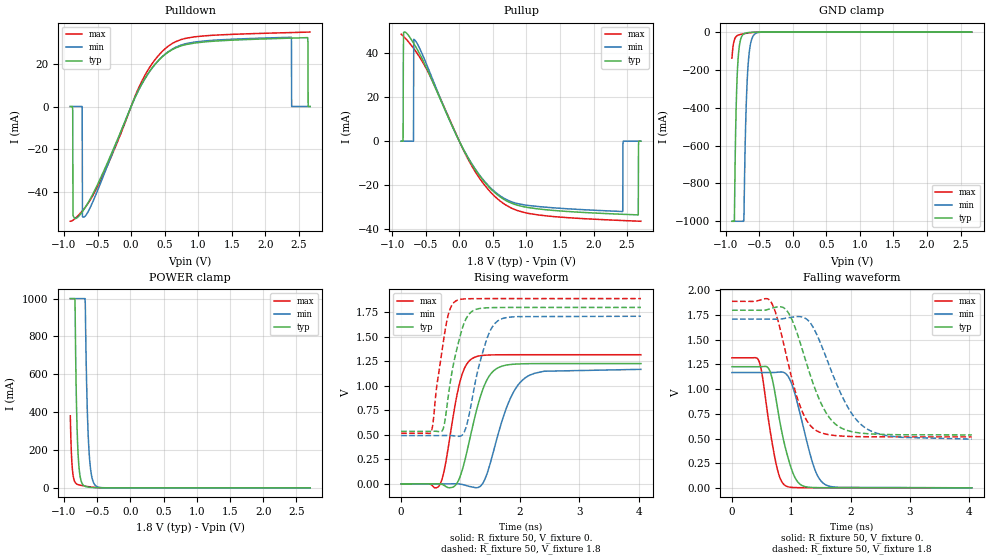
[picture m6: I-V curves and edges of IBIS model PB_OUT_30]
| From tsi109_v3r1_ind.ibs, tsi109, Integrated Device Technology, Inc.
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[Model]   PB_OUT_30
Model_type  Output
Polarity   Non-Inverting
Enable   Active-High
|   typ   min   max
|C_comp_off 3.714p 3.449p 3.979p
|C_comp_on 4.306p 3.81p 4.757p
C_comp 4.01p 3.63p 4.368p
Vinl  =   0.300v
Vinh  =   1.500v
Vmeas =   0.9000V
Cref  =   1.0pF
Rref  =   50.0000
Vref  =   0.0V
[Model Spec]
[Temperature Range]   25   125   -40
[Voltage Range] 1.8 1.71 1.89
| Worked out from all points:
|   slope of the pulldown table from 0 to 0.27 V, typ, clamps not added: 16.6 ohm
|   slope of the pullup table from 0 to 0.27 V, typ, clamps not added: 18.8 ohm
|   GND clamp passes 1 mA (typ) near -0.59 V on its own axis
|   POWER clamp passes 1 mA (typ) near -0.54 V on its own axis
|   rising waveform, R_fixture 50, V_fixture 0.: 20-80 % time 312ps typ, 380ps min, 232ps max; typ from 0 V to 1.23 V
|   rising waveform, R_fixture 50, V_fixture 1.8: 20-80 % time 240ps typ, 282ps min, 190ps max; typ from 0.536 V to 1.8 V
|   falling waveform, R_fixture 50, V_fixture 0.: 20-80 % time 255ps typ, 300ps min, 205ps max; typ from 1.23 V to 0 V
|   falling waveform, R_fixture 50, V_fixture 1.8: 20-80 % time 451ps typ, 545ps min, 363ps max; typ from 1.8 V to 0.536 V
[Pulldown]
-905.9mV  0A         0A         -53.93mA
-866.2mV  -51.03mA   0A         -53.42mA
-826.5mV  -52.6mA    0A         -52.37mA
-728.9mV  -49.53mA   0A         -49.13mA
-725.3mV  -49.37mA   -51.66mA   -48.99mA
-696.4mV  -48.04mA   -51.83mA   -47.86mA
661.7mV   27.52mA    27.83mA    30.46mA
2.388V    32.15mA    32.55mA    34.76mA
2.392V    32.16mA    0A         34.77mA
2.63V     32.37mA    0A         34.97mA
2.638V    0A         0A         34.98mA
2.667V    0A         0A         35.01mA
[Pullup]
-866.5mV  0A         0A         48.72mA
-837.6mV  0A         0A         47.94mA
-830.4mV  49.49mA    0A         47.72mA
-815.9mV  49.71mA    0A         47.26mA
-682.3mV  44.71mA    0A         42.34mA
-678.7mV  44.53mA    46.42mA    42.2mA
769.8mV   -28.13mA   -27.5mA    -30.36mA
2.435V    -33.28mA   -32.01mA   -36.12mA
2.442V    -33.29mA   0A         -36.13mA
2.666V    -33.56mA   0A         -36.41mA
2.67V     -1.866mA   0A         -36.41mA
2.706V    0A         0A         -36.46mA
[GND Clamp]
-905.9mV  -1A        -1A        -137.9mA
-870.3mV  -1A        -1A        -41.43mA
-846.6mV  -441.9mA   -1A        -24.54mA
-818.8mV  -164.5mA   -1A        -17.08mA
-787.2mV  -54.7mA    -1A        -13.21mA
-735.7mV  -11.66mA   -1A        -9.248mA
-727.8mV  -9.573mA   -983.7mA   -8.719mA
-700.1mV  -5.335mA   -460.2mA   -6.983mA
-672.3mV  -3.348mA   -211.4mA   -5.421mA
-632.8mV  -1.857mA   -68.65mA   -3.514mA
-569.4mV  -685.4uA   -11.35mA   -1.391mA
2.667V    0A         0A         0A
[Power Clamp]
-905.9mV  1A         1A         380.5mA
-878.2mV  1A         1A         113.3mA
-835mV    992.8mA    1A         29.9mA
-813.4mV  448.2mA    1A         21.21mA
-788.7mV  179.3mA    1A         16.86mA
-699.3mV  10.92mA    1A         10.05mA
-680.8mV  7.495mA    977.8mA    8.969mA
-662.3mV  5.499mA    579.6mA    7.938mA
-625.2mV  3.317mA    200.9mA    6.022mA
-585.1mV  1.988mA    63.4mA     4.19mA
-520.4mV  744.8uA    9.906mA    1.885mA
2.706V    0A         0A         0A
[Ramp]
dV/dt_r .737/312.486p .701/380.002p .791/232.014p
dV/dt_f .758/450.715p .73/545.704p .824/362.761p
[Rising Waveform]
R_fixture = 50
V_fixture = 0.
0s        0V         0V         0V
650ps     555.7uV    -23.99uV   -9.787mV
950ps     16.08mV    470uV      934.5mV
1.07ns    232.3mV    -11.99mV   1.183V
1.23ns    652.4mV    -35.49mV   1.29V
1.39ns    985.6mV    21.28mV    1.311V
1.53ns    1.136V     273.6mV    1.316V
1.81ns    1.215V     830mV      1.317V
2.09ns    1.226V     1.081V     1.318V
4.04ns    1.228V     1.168V     1.318V
[Rising Waveform]
R_fixture = 50
V_fixture = 1.8
V_fixture_min = 1.71
V_fixture_max = 1.89
0s        536.1mV    492.7mV    516.3mV
510ps     536.3mV    492.7mV    533.1mV
710ps     564.5mV    493mV      1.446V
810ps     965.1mV    493.8mV    1.758V
930ps     1.354V     487.5mV    1.869V
1.05ns    1.622V     513.9mV    1.886V
1.15ns    1.736V     719.1mV    1.889V
1.41ns    1.795V     1.414V     1.89V
1.63ns    1.799V     1.663V     1.89V
4.04ns    1.8V       1.71V      1.89V
[Falling Waveform]
R_fixture = 50
V_fixture = 0.
0s        1.228V     1.168V     1.318V
460ps     1.228V     1.168V     1.277V
660ps     1.146V     1.168V     516.3mV
780ps     762.9mV    1.172V     152.7mV
900ps     405.5mV    1.16V      22.2mV
1ns       195.5mV    1.064V     4.98mV
1.12ns    51.47mV    817mV      1.946mV
1.38ns    3.13mV     212.7mV    558.5uV
1.56ns    1.376mV    37.03mV    240.4uV
4.04ns    0V         9.409uV    0V
[Falling Waveform]
R_fixture = 50
V_fixture = 1.8
V_fixture_min = 1.71
V_fixture_max = 1.89
0s        1.8V       1.71V      1.89V
660ps     1.819V     1.71V      1.881V
780ps     1.835V     1.709V     1.683V
980ps     1.743V     1.727V     1.178V
1.19ns    1.391V     1.73V      765mV
1.42ns    971.5mV    1.565V     580.9mV
1.74ns    647.4mV    1.085V     529.7mV
2ns       572.1mV    769.5mV    520.6mV
2.24ns    550.8mV    610.5mV    517.9mV
4.04ns    536.1mV    493.7mV    516.3mV
